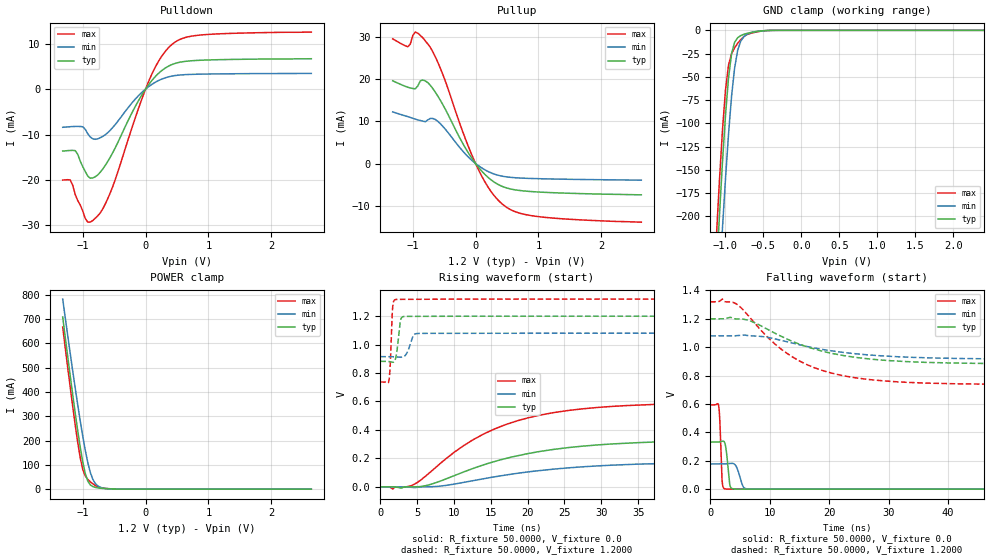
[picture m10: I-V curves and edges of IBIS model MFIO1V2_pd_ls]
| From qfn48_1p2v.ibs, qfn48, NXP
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[Model] MFIO1V2_pd_ls
|   Model MFIO1V2_pd_ls
| This model was characterised for following simulation conditions:
| External (pad) voltage:
|   - Typ: 1.2V,   - Min: 1.08V,   - Max: 1.32V
| Library cells for typ/min/max conditions are connected as defined below:
|  IO - External Pad
|  A - Core Input
|  EN - Output Buffer Enable
|  BOOST - vdde
|  EHS - gnd
|  ENZI - vdd
|  EPD - vdd
|  EPUN - vdd
|  ZI - NC
|  ZIF - NC
|  gnd - gnd
|  gnde - gnde
|  vdd - vdd
|  vdde - vdde
| All other pins connected to ground
Model_type I/O
Polarity   Non-Inverting
Enable   Active-Low
Vinl =   0.3600V
Vinh =   0.8400V
Vmeas =  0.6000V
Cref =   20.0000F
Rref =   1.0000M
Vref =   0.0V
C_comp   1.6368pF   1.5495pF   1.7159pF
|C_comp_pullup   0.8309pF   0.8676pF   0.7830pF
|C_comp_pulldown   0.5929pF   0.6311pF   0.5574pF
[Model Spec]
| variable   typ   min   max
Vinh   0.3600V   0.3240V   0.3960V
Vinl   0.8400V   0.7560V   0.9240V
Vmeas   0.6000V   0.5400V   0.6600V
[Temperature Range]   25.0000   0.1250k   -40.0000
[Voltage Range]   1.2000V   1.0800V   1.3200V
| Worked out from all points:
|   slope of the pulldown table from 0 to 0.18 V, typ, clamps not added: 58.2 ohm
|   slope of the pullup table from 0 to 0.18 V, typ, clamps not added: 59.4 ohm
|   GND clamp passes 1 mA (typ) near -0.56 V on its own axis
|   POWER clamp passes 1 mA (typ) near -0.54 V on its own axis
|   rising waveform, R_fixture 50.0000, V_fixture 0.0: 20-80 % time 14.4ns typ, 16.1ns min, 12.2ns max; typ from 0 V to 0.331 V
|   rising waveform, R_fixture 50.0000, V_fixture 1.2000: 20-80 % time 407ps typ, 669ps min, 259ps max; typ from 0.882 V to 1.2 V
|   falling waveform, R_fixture 50.0000, V_fixture 0.0: 20-80 % time 465ps typ, 791ps min, 298ps max; typ from 0.331 V to 0 V
|   falling waveform, R_fixture 50.0000, V_fixture 1.2000: 20-80 % time 12.6ns typ, 13.9ns min, 10.9ns max; typ from 1.2 V to 0.882 V
[Pulldown]
|Voltage   I(typ)   I(min)   I(max)
-1.32V    -13.65mA   -8.413mA   -20.02mA
-1.2V     -13.51mA   -8.286mA   -20.01mA
-1.12V    -13.55mA   -8.228mA   -23.23mA
-920mV    -19.16mA   -9.849mA   -29.29mA
-720mV    -18.27mA   -10.7mA    -27.21mA
-520mV    -13.92mA   -8.406mA   -21.33mA
-160mV    -3.727mA   -2.148mA   -6.154mA
80mV      1.535mA    840.4uA    2.681mA
280mV     4.299mA    2.312mA    7.674mA
480mV     5.684mA    2.989mA    10.42mA
960mV     6.383mA    3.3mA      11.99mA
2.64V     6.67mA     3.446mA    12.53mA
[Pullup]
|Voltage   I(typ)   I(min)   I(max)
-1.32V    19.64mA    12.26mA    29.6mA
-1.08V    18.12mA    11.13mA    27.73mA
-960mV    17.74mA    10.54mA    31.21mA
-840mV    19.83mA    10.07mA    29.84mA
-720mV    18.57mA    10.71mA    27.56mA
-520mV    13.94mA    8.794mA    21.09mA
-200mV    4.663mA    2.883mA    7.362mA
40mV      -771.3uA   -452.7uA   -1.28mA
240mV     -3.804mA   -2.171mA   -6.507mA
480mV     -5.732mA   -3.143mA   -10.26mA
1.04V     -6.794mA   -3.614mA   -12.68mA
2.64V     -7.439mA   -3.951mA   -13.93mA
[GND_clamp]
|Voltage   I(typ)   I(min)   I(max)
-1.32V    -596.2mA   -647.7mA   -564.2mA
-1.12V    -261.7mA   -329.6mA   -222.8mA
-1.08V    -200.1mA   -270.2mA   -162.2mA
-1.04V    -142.4mA   -213.4mA   -108mA
-1V       -91.66mA   -160.1mA   -64.4mA
-960mV    -51.26mA   -111.8mA   -37.36mA
-920mV    -25.17mA   -71.04mA   -25.19mA
-880mV    -12.89mA   -40.68mA   -18.85mA
-800mV    -5.7mA     -11.79mA   -10.05mA
-680mV    -2.586mA   -2.926mA   -3.538mA
-440mV    -160.8uA   -186.1uA   -197.3uA
2.64V     0A         0A         0A
[POWER_clamp]
|Voltage   I(typ)   I(min)   I(max)
-1.32V    708.1mA    782.2mA    666.5mA
-1.2V     465.5mA    558mA      418.6mA
-1.12V    311.6mA    414.8mA    262.8mA
-1.04V    171.5mA    279.6mA    128.1mA
-1V       111.7mA    217mA      80.3mA
-960mV    64.07mA    159.3mA    53.87mA
-920mV    33.02mA    108.9mA    40.24mA
-880mV    17.44mA    68.44mA    30.42mA
-840mV    10.78mA    40.19mA    22.06mA
-760mV    5.295mA    13.21mA    9.362mA
-440mV    235.7uA    303.1uA    277.6uA
2.64V     0A         0A         0A
[Ramp]
| variable   typ   min   max
dV/dt_r  0.1988/14.4182n   0.1066/16.0994n   0.3561/12.2272n
dV/dt_f  0.1904/12.5990n   98.7976m/13.9393n   0.3496/10.8773n
R_load = 50.0000
[Rising Waveform]
R_fixture= 50.0000
V_fixture= 0.0
V_fixture_min= 0.0
V_fixture_max= 0.0
|time   V(typ)   V(min)   V(max)
0s        1.234nV    117.7nV    49.88pV
1.703ns   71.76uV    73.64uV    -16.38mV
4.491ns   -508.6uV   -4.553mV   14.43mV
6.803ns   16.6mV     466.2uV    104mV
11.25ns   103.4mV    30.34mV    287.3mV
17ns      198.6mV    82.88mV    437mV
21.68ns   248.8mV    114.7mV    504mV
27.08ns   283.9mV    139.4mV    546.2mV
45.08ns   324.1mV    170.7mV    587.6mV
100ns     331.4mV    177.6mV    593.5mV
[Rising Waveform]
R_fixture= 50.0000
V_fixture= 1.2000
V_fixture_min= 1.0800
V_fixture_max= 1.3200
|time   V(typ)   V(min)   V(max)
0s        882mV      914.8mV    736.7mV
1.166ns   880.6mV    915mV      743.3mV
1.362ns   878.7mV    915.1mV    866.2mV
1.679ns   875.4mV    914.4mV    1.262V
2.123ns   911.6mV    912.8mV    1.317V
2.75ns    1.171V     910.6mV    1.317V
3.318ns   1.198V     919.4mV    1.317V
4.487ns   1.198V     1.062V     1.317V
5.341ns   1.198V     1.078V     1.318V
100ns     1.199V     1.079V     1.319V
[Falling Waveform]
R_fixture= 50.0000
V_fixture= 0.0
V_fixture_min= 0.0
V_fixture_max= 0.0
|time   V(typ)   V(min)   V(max)
0s        331.4mV    177.7mV    593.5mV
1.413ns   331.7mV    177.7mV    587.2mV
1.613ns   333.4mV    177.6mV    476.8mV
2.005ns   337.9mV    177.5mV    51.91mV
2.549ns   308mV      178.4mV    1.374mV
3.304ns   28.73mV    181.4mV    678.1uV
4.032ns   1.028mV    177.2mV    787.5uV
5.55ns    562.9uV    16.22mV    578uV
6.566ns   523.8uV    962.4uV    434.3uV
100ns     11.26nV    159.9nV    8.884nV
[Falling Waveform]
R_fixture= 50.0000
V_fixture= 1.2000
V_fixture_min= 1.0800
V_fixture_max= 1.3200
|time   V(typ)   V(min)   V(max)
0s        1.199V     1.079V     1.319V
2.013ns   1.199V     1.079V     1.339V
4.52ns    1.199V     1.081V     1.301V
6.656ns   1.186V     1.08V      1.209V
10.75ns   1.101V     1.06V      1.027V
14.75ns   1.025V     1.019V     908.4mV
18.67ns   973.5mV    985.7mV    838.3mV
24.41ns   928.3mV    953.8mV    784.4mV
42.48ns   887.2mV    920mV      741.4mV
100ns     882mV      914.8mV    736.7mV
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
